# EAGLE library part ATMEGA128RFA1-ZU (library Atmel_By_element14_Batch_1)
8-bit Microcontroller
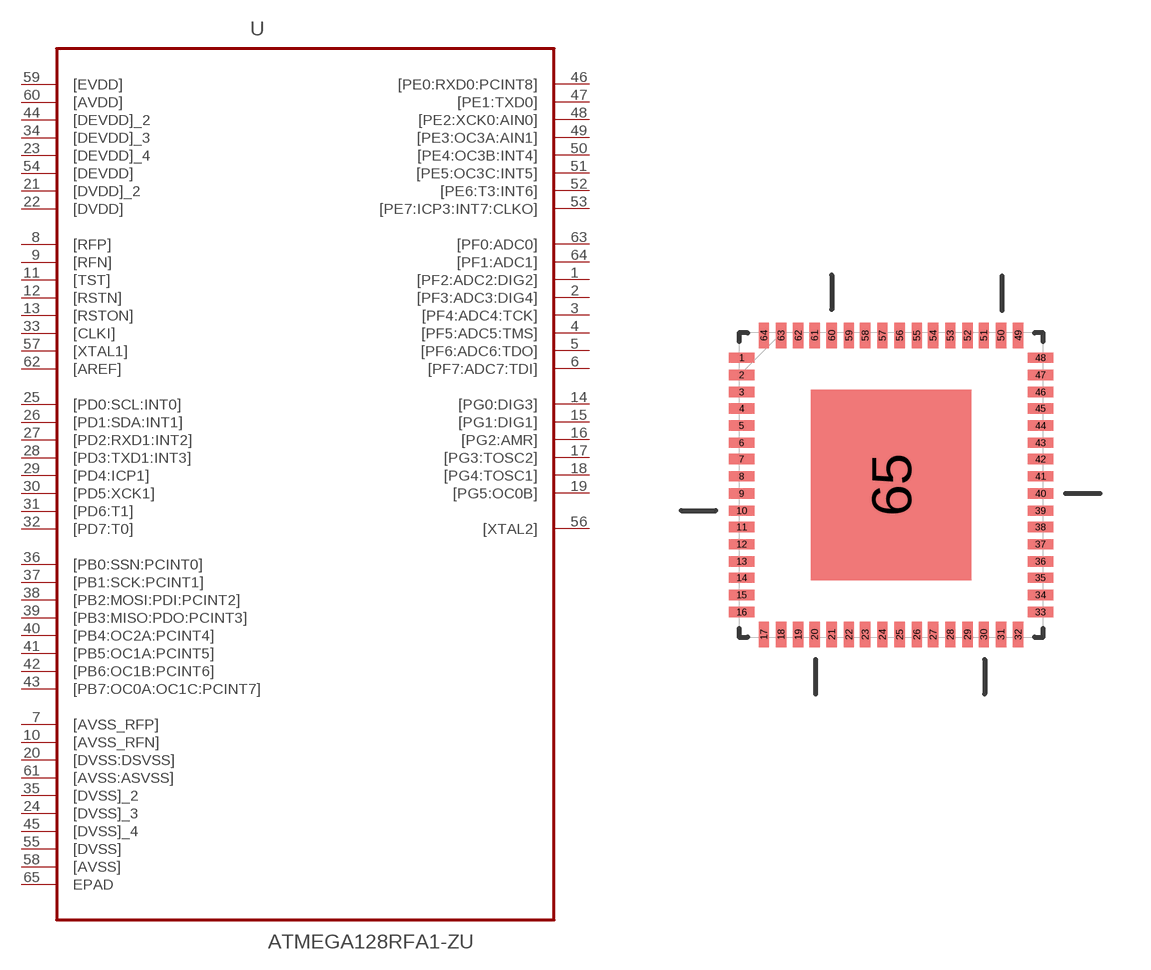
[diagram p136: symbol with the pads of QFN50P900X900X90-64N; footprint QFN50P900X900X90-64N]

Designator prefix U

## ATMEGA128RFA1-ZU (DESCRIPTION: 8-bit Microcontroller; MPN: ATMEGA128RFA1-ZU; OC_FARNELL: 1841596; OC_NEWARK: -; PACKAGE: QFN-64; SUPPLIER: Atmel)  [QFN50P900X900X90-64N]
1  [PF2:ADC2:DIG2]
2  [PF3:ADC3:DIG4]
3  [PF4:ADC4:TCK]
4  [PF5:ADC5:TMS]
5  [PF6:ADC6:TDO]
6  [PF7:ADC7:TDI]
7  [AVSS_RFP]  pwr
8  [RFP]  in
9  [RFN]  in
10  [AVSS_RFN]  pwr
11  [TST]  in
12  [RSTN]  in
13  [RSTON]  in
14  [PG0:DIG3]
15  [PG1:DIG1]
16  [PG2:AMR]
17  [PG3:TOSC2]
18  [PG4:TOSC1]
19  [PG5:OC0B]
20  [DVSS:DSVSS]  pwr
21  [DVDD]_2  pwr
22  [DVDD]  pwr
23  [DEVDD]_4  pwr
24  [DVSS]_3  pwr
25  [PD0:SCL:INT0]
26  [PD1:SDA:INT1]
27  [PD2:RXD1:INT2]
28  [PD3:TXD1:INT3]
29  [PD4:ICP1]
30  [PD5:XCK1]
31  [PD6:T1]
32  [PD7:T0]
33  [CLKI]  in
34  [DEVDD]_3  pwr
35  [DVSS]_2  pwr
36  [PB0:SSN:PCINT0]
37  [PB1:SCK:PCINT1]
38  [PB2:MOSI:PDI:PCINT2]
39  [PB3:MISO:PDO:PCINT3]
40  [PB4:OC2A:PCINT4]
41  [PB5:OC1A:PCINT5]
42  [PB6:OC1B:PCINT6]
43  [PB7:OC0A:OC1C:PCINT7]
44  [DEVDD]_2  pwr
45  [DVSS]_4  pwr
46  [PE0:RXD0:PCINT8]
47  [PE1:TXD0]
48  [PE2:XCK0:AIN0]
49  [PE3:OC3A:AIN1]
50  [PE4:OC3B:INT4]
51  [PE5:OC3C:INT5]
52  [PE6:T3:INT6]
53  [PE7:ICP3:INT7:CLKO]
54  [DEVDD]  pwr
55  [DVSS]  pwr
56  [XTAL2]  out
57  [XTAL1]  in
58  [AVSS]  pwr
59  [EVDD]  pwr
60  [AVDD]  pwr
61  [AVSS:ASVSS]  pwr
62  [AREF]  in
63  [PF0:ADC0]
64  [PF1:ADC1]
65  EPAD  pas

## Footprint QFN50P900X900X90-64N (pad centres in mm)
smd 0.762 x 0.305: 1 -4.42,3.759; 2 -4.42,3.251; 3 -4.42,2.743; 4 -4.42,2.261; 5 -4.42,1.753; 6 -4.42,1.245; 7 -4.42,0.762; 8 -4.42,0.254; 9 -4.42,-0.254; 10 -4.42,-0.762; 11 -4.42,-1.245; 12 -4.42,-1.753; 13 -4.42,-2.261; 14 -4.42,-2.743; 15 -4.42,-3.251; 16 -4.42,-3.759; 33 4.42,-3.759; 34 4.42,-3.251; 35 4.42,-2.743; 36 4.42,-2.261; 37 4.42,-1.753; 38 4.42,-1.245; 39 4.42,-0.762; 40 4.42,-0.254; 41 4.42,0.254; 42 4.42,0.762; 43 4.42,1.245; 44 4.42,1.753; 45 4.42,2.261; 46 4.42,2.743; 47 4.42,3.251; 48 4.42,3.759
smd 0.305 x 0.762: 17 -3.759,-4.42; 18 -3.251,-4.42; 19 -2.743,-4.42; 20 -2.261,-4.42; 21 -1.753,-4.42; 22 -1.245,-4.42; 23 -0.762,-4.42; 24 -0.254,-4.42; 25 0.254,-4.42; 26 0.762,-4.42; 27 1.245,-4.42; 28 1.753,-4.42; 29 2.261,-4.42; 30 2.743,-4.42; 31 3.251,-4.42; 32 3.759,-4.42; 49 3.759,4.42; 50 3.251,4.42; 51 2.743,4.42; 52 2.261,4.42; 53 1.753,4.42; 54 1.245,4.42; 55 0.762,4.42; 56 0.254,4.42; 57 -0.254,4.42; 58 -0.762,4.42; 59 -1.245,4.42; 60 -1.753,4.42; 61 -2.261,4.42; 62 -2.743,4.42; 63 -3.251,4.42; 64 -3.759,4.42
smd 4.75 x 5.639: 65 0,0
